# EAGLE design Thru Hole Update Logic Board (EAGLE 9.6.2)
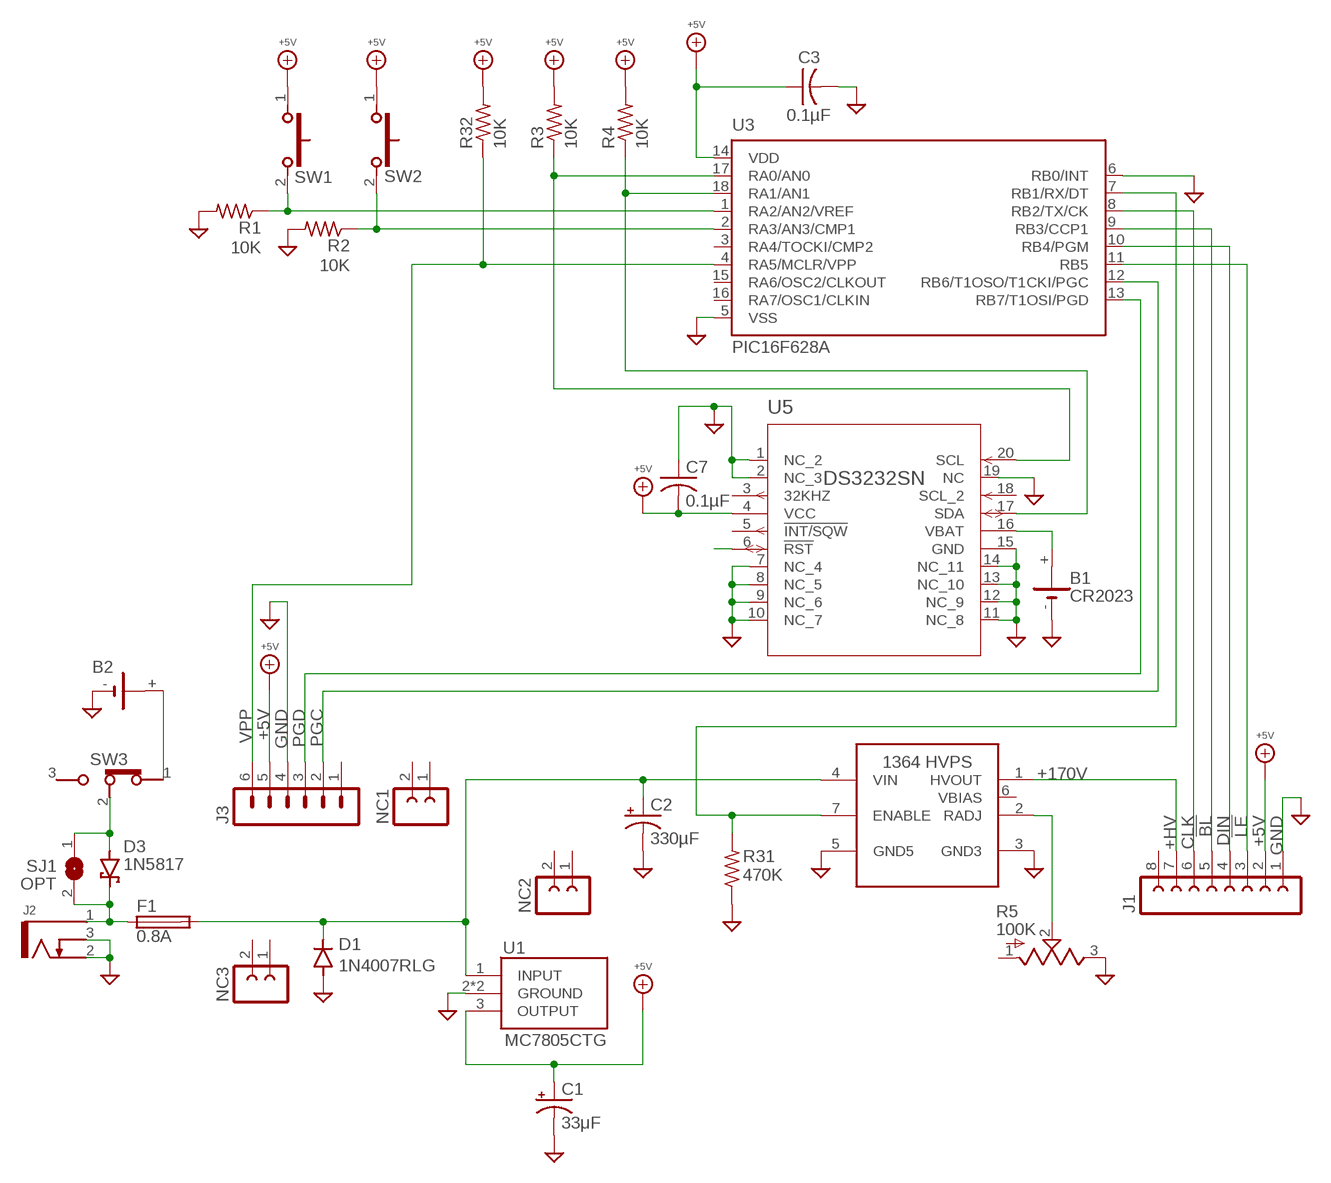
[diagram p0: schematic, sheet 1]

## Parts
B1  CR2023  BATTERY  [103]
B2  BATTERYWIRE_ATTACH  BATTERY1291  [1291]
C1  33μF  CPOL-USE2-5  [E2-5]
C2  330µF  CPOL-USE3.5-8  [E3,5-8]
C3  0.1µF  C-US  [C025-040X050]
C7  0.1µF  C-USC0805  [C0805]
D1  1N4007RLG  RECTIFIER  [DO41-7]
D3  1N5817  SCHOTTKY  [DO41-7]
F1  0.8A  FUSE  [5X20MM]
J1  FE08  [FE08]
J2  KLDX-0202-B  [KDLX-0202-X]
J3  MA06  [MA06]
NC1  FE02  [FE02]
NC2  FE02  [FE02]
NC3  FE02  [FE02]
R1  10K  R-US0207/10  [0207/10]
R2  10K  R-US0207/10  [0207/10]
R3  10K  R-US0207/10  [0207/10]
R4  10K  R-US0207/10  [0207/10]
R5  100K  R-US_TRIM  [PV37W]
R31  470K  R-US0207/10  [0207/10]
R32  10K  R-US0207/10  [0207/10]
SJ1  OPT  SJ  [SJ]
SW1  FSMRA4JH04  SWITCH_PUSH_SPST_(ON)  [FSMRA4JH]
SW2  FSMRA4JH04  SWITCH_PUSH_SPST_(ON)  [FSMRA4JH]
SW3  5MS1S102AM6QES  SWITCH_SLIDE_SPDT_ON  [SLIDE_SPDT_MINI]
U1  MC7805CTG  [TO-220-3_RA]
U2  1364-HVPS-H  [1364-HVPS-H]
U3  PIC16F628A  PIC16F628P  [DIP-18]
U5  DS3232SN  [SOIC-20]

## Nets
!BL!: J1.5 U3.9(RB3/CCP1)
!LE!: J1.3 U3.11(RB5)
+5V: C1.+ C3.1 C7.2 J1.2 J3.5 R3.2 R4.2 R32.2 SW1.1 SW2.1 U1.3(OUTPUT) U3.14(VDD) U5.4(VCC)
+9V: D3.C F1.1A F1.1B J2.1 SJ1.2
+9V_1: C2.+ D1.C F1.2A F1.2B U1.1(INPUT) U2.4(VIN)
+9V_2: D3.A SJ1.1 SW3.2(COM)
+9V_4: B2.+ SW3.1(POS_1)
+HV: J1.7 U2.1(HVOUT)
BAT: B1.+ U5.16(VBAT)
CLK: J1.6 U3.8(RB2/TX/CK)
DIN: J1.4 U3.10(RB4/PGM)
ENABLE: R31.2 U2.7(ENABLE) U3.7(RB1/RX/DT)
GND: B1.- B2.- C1.- C2.- C3.2 C7.1 D1.A J1.1 J2.2 J2.3 J3.4 R1.2 R2.2 R5.3 R31.1 U1.2(GROUND) U1.2_1(GROUND) U2.3(GND3) U2.5(GND5) U3.5(VSS) U3.6(RB0/INT) U5.1(NC_2) U5.2(NC_3) U5.7(NC_4) U5.8(NC_5) U5.9(NC_6) U5.10(NC_7) U5.11(NC_8) U5.12(NC_9) U5.13(NC_10) U5.14(NC_11) U5.15(GND) U5.19(NC)
MYSTERY_3: U5.6(!RST)
PGC: J3.2 U3.12(RB6/T1OSO/T1CKI/PGC)
PGD: J3.3 U3.13(RB7/T1OSI/PGD)
RADJ: R5.2 U2.2(RADJ)
SCL: R3.1 U3.17(RA0/AN0) U5.20(SCL)
SDA: R4.1 U3.18(RA1/AN1) U5.17(SDA)
SW1: R1.1 SW1.2 U3.1(RA2/AN2/VREF)
SW2: R2.1 SW2.2 U3.2(RA3/AN3/CMP1)
VPP: J3.6 R32.1 U3.4(RA5/MCLR/VPP)
Unconnected: J1.8 J3.1 NC1.1 NC1.2 NC2.1 NC2.2 NC3.1 NC3.2 R5.1 SW3.3(POS_2) U2.6(VBIAS) U3.3(RA4/TOCKI/CMP2) U3.15(RA6/OSC2/CLKOUT) U3.16(RA7/OSC1/CLKIN) U5.3(32KHZ) U5.5(!INT/SQW) U5.18(SCL_2)

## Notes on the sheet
- +170V

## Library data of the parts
B1 B2 = My Imported Components:BATTERY: LI BATTERY Varta
C1 C2 = My Imported Components:CPOL-US
C3 = My Imported Components:C-US
C7 = rcl:C-US: CAPACITOR, American symbol; SPICEPREFIX: C
D1 = My Imported Components:RECTIFIER
D3 = My Imported Components:SCHOTTKY
F1 = My Imported Components:FUSE
J1 = My Imported Components:FE08: FEMALE HEADER; OC_FARNELL: unknown; OC_NEWARK: unknown
J2 = My Imported Components:KLDX-0202-B: https://www.mouser.com/datasheet/2/222/KLDX_0202-334781.pdf
J3 = My Imported Components:MA06: PIN HEADER; OC_FARNELL: unknown; OC_NEWARK: unknown
NC1-NC3 = My Imported Components:FE02: FEMALE HEADER
R1-R4 R31 R32 = My Imported Components:R-US: RESISTOR, American symbol; SPICEPREFIX: R
R5 = My Imported Components:R-US_TRIM: Res Cermet Trimmer 1M Ohm 10% 1/4W 12(Elec)Turn 1.8mm (6.4 X 4 X 7.7mm) Pin Thru-Hole Bulk Check prices; AVAILABILITY: Good; DESCRIPTION: 100 kOhms 0.25W, 1/4W PC Pins Through Hole Trimmer Potentiometer Cermet 12 Turn Top Adjustment; MF: Bourns; MP: PV37W104C01B00; PACKAGE: 3224X Bourns; PRICE: None; PURCHASE-URL: https://pricing.snapeda.com/search/part/PV37W104C01B00/?ref=eda
SJ1 = jumper:SJ: SMD solder JUMPER
SW1 SW2 = My Imported Components:SWITCH_PUSH_SPST_(ON)
SW3 = My Imported Components:SWITCH_SLIDE_SPDT_ON
U1 = My Imported Components:MC7805CTG: Voltage regulator,MC7805CT 5V 1A ON Semiconductor MC7805CTG, Single Linear Voltage Regulator, 1A 5 V, +/-4%, 3-Pin TO-220 Source: Datasheet; ARROW_PART_NUMBER: MC7805CTG; ARROW_PRICE-STOCK: https://www.arrow.com/en/products/mc7805ctg/on-semiconductor; DESCRIPTION: Voltage regulator,MC7805CT 5V 1A ON Semiconductor MC7805CTG, Single Linear Voltage Regulator, 1A 5 V, +/-4%, 3-Pin TO-220; HEIGHT: 4.82mm; MANUFACTURER_NAME: ON Semiconductor; MANUFACTURER_PART_NUMBER: MC7805CTG; MOUSER_PART_NUMBER: 863-MC7805CTG; MOUSER_PRICE-STOCK: https://www.mouser.co.uk/ProductDetail/ON-Semiconductor/MC7805CTG/?qs=%252B9%2Fcbd0IE0SRQQJXyw%252B9hQ%3D%3D
U2 = My Imported Components:1364-HVPS-H: https://www.shop-tes.com/content/Datasheets/8002K.pdf
U3 = My Imported Components:PIC16F62*: FLASH-Based 8-Bit CMOS Microcontroller Source: http://ww1.microchip.com/downloads/en/DeviceDoc/40300C.pdf; MF: MICROCHIP; MPN: PIC16F628-04I/P; OC_FARNELL: 9760407; OC_NEWARK: 19C7272
U5 = My Imported Components:DS3232SN; BUILT_BY: EMA_UL_Team; MANUFACTURER_PART_NUMBER: ds3232sn#; SOURCELIBRARY: Maxim_2009-12-17_1; VENDOR: Maxim Integrated Products

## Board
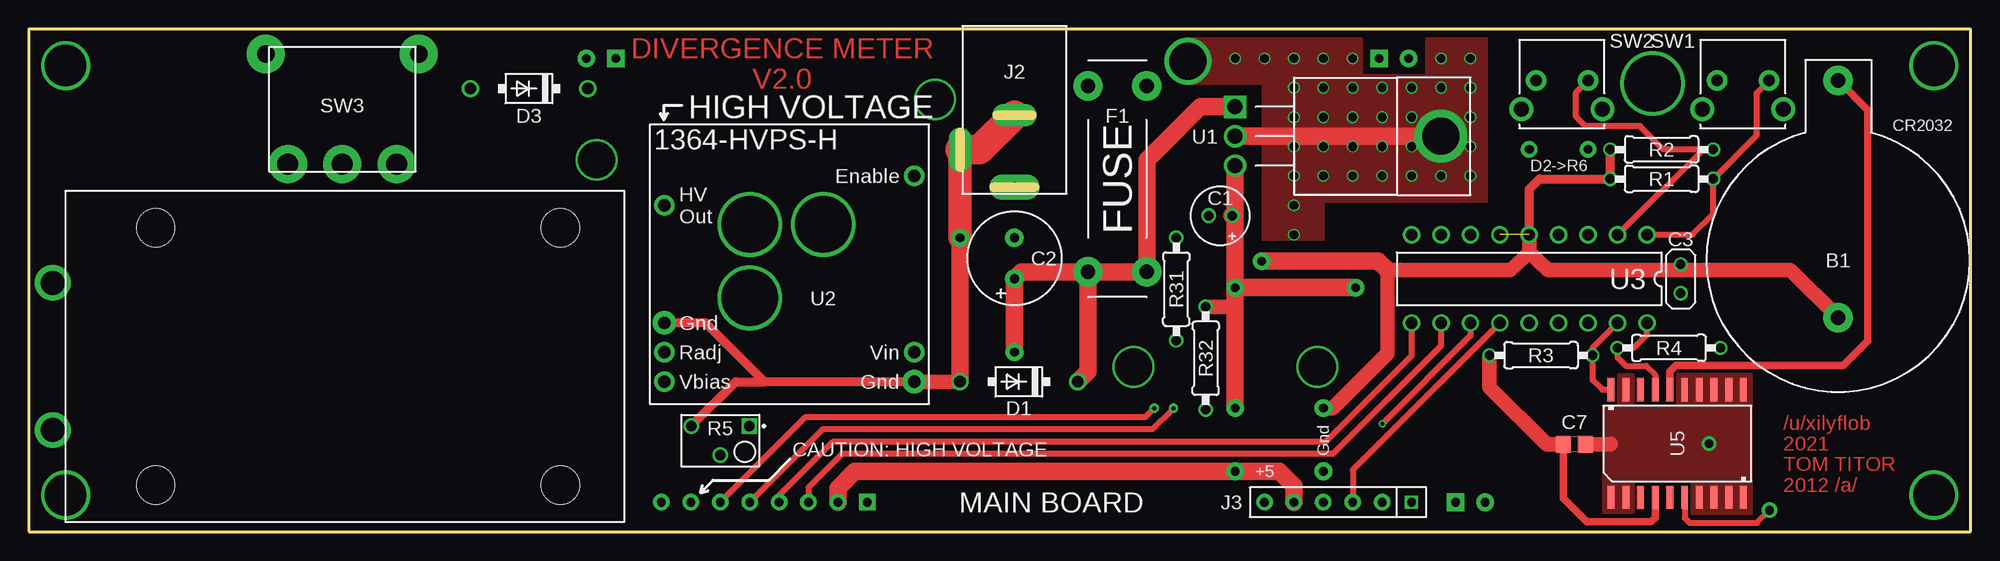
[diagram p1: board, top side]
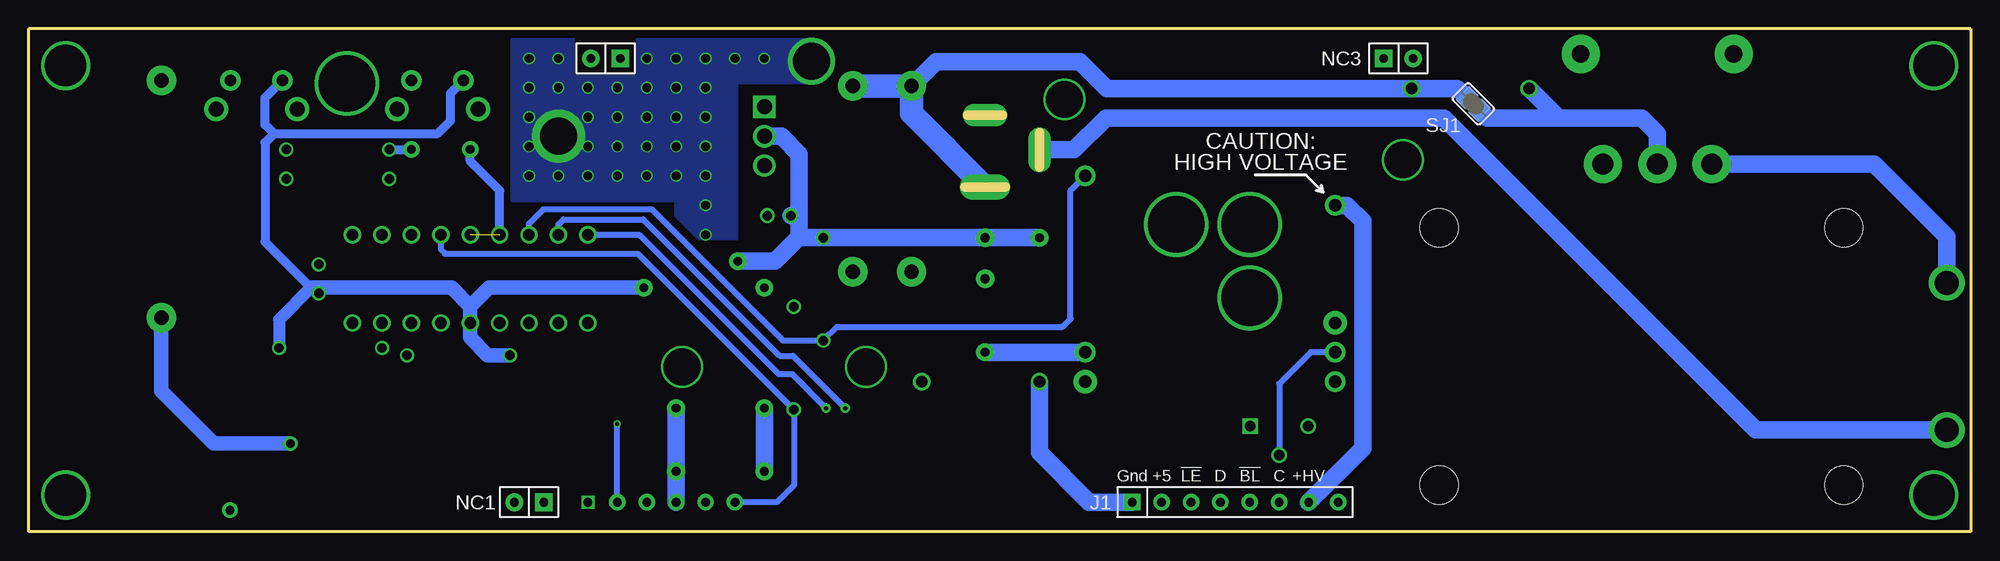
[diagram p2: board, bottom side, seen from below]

Size 167.64 x 43.43 mm. Coordinates in mm from the lower left corner, seen from the top.
Outline: 0,0 167.64,0 167.64,43.43 0,43.43 0,0
Copper layers (1*16): Top 0.035559375mm / dielectric 1.6mm / Bottom 0.035559375mm
Design rules "oshpark-2layer *": minimum track width 6mil, minimum drill 10mil, track to track 6mil, track to pad 6mil, pad to pad 6mil, via to via 6mil, smd to smd 6mil, copper to edge 15mil, drill to drill 6mil, minimum pad ring 5mil, minimum via ring 5mil, stop-mask expansion 2.5mil, vias tented up to drill 0mil, thermal gap 10mil

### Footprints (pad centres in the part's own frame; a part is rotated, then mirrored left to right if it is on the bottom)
103 = drill 1.27 pad 2.54: + 0,0; - 0,-20.498
1291 = drill 2.057: + 8.89,-6.35; - 8.89,6.35 | hole 3.302: -34.925,11.113; 0,11.113; 0,-11.113; -34.925,-11.113
E2-5 = drill 0.813 pad 1.27: + -1.016,0; - 1.016,0
E3,5-8 = drill 0.813 pad 1.6: + -1.778,0; - 1.778,0
C025-040X050 = drill 0.813: 1 -1.25,0; 2 1.25,0
C0805 = smd 1.3 x 1.5: 1 -0.95,0; 2 0.95,0
DO41-7 = drill 1: A 5.08,0; C -5.08,0
5X20MM = drill 1.245 pad 2.54: 1A -8.026,2.54; 1B -8.026,-2.54; 2A 8.026,2.54; 2B 8.026,-2.54
FE08 = drill 0.75 pad 1.422 square: 1 -8.89,0 | drill 0.75 pad 1.422: 2 -6.35,0; 3 -3.81,0; 4 -1.27,0; 5 1.27,0; 6 3.81,0; 7 6.35,0; 8 8.89,0
KDLX-0202-X = drill 0.8 pad 2.184 long: 1 13.9,0 | drill 0.8 pad 1.93 long: 2 7.7,0; 3 10.7,-4.7
MA06 = drill 0.75 square: 1 -6.35,0 | drill 0.75 pad 1.422: 2 -3.81,0; 3 -1.27,0; 4 1.27,0; 5 3.81,0; 6 6.35,0
FE02 = drill 0.75 pad 1.524 square: 1 -1.27,0 | drill 0.75 pad 1.524: 2 1.27,0
0207/10 = drill 0.813: 1 -4.445,0; 2 4.445,0
PV37W = drill 0.9 square: 1 -2.5,-1.25 | drill 0.9: 2 0,1.25; 3 2.5,-1.25
SJ = smd 1.168 x 1.6: 1 -0.762,0; 2 0.762,0
FSMRA4JH = drill 0.991 pad 1.753: 1 4.496,0; 2 0,0 | drill 1.295 pad 2.057: 3 -1.245,2.489; 4 5.766,2.489
SLIDE_SPDT_MINI = drill 1.8 pad 3.302: 1 -4.699,0; 2 0,0; 3 4.699,0 | drill 1.5 pad 3.302: P$4 -6.604,9.525; P$5 6.604,9.525
TO-220-3_RA = drill 1.29 pad 1.935 square: 1 0,0 | drill 1.29 pad 1.935: 2 2.54,0; 3 5.08,0 | drill 3.175 pad 4.572: 2_1 2.54,17.78
1364-HVPS-H = drill 1.067 pad 1.778: 1 1.27,17.145; 2 1.27,4.445; 4 22.86,4.445; 6 1.27,1.905; 7 22.86,19.685 | drill 1.067 pad 2.032: 3 1.27,6.985; 5 22.86,1.905
DIP-18 = drill 1: 1 -10.16,-3.81; 2 -7.62,-3.81; 3 -5.08,-3.81; 4 -2.54,-3.81; 5 0,-3.81; 6 2.54,-3.81; 7 5.08,-3.81; 8 7.62,-3.81; 9 10.16,-3.81; 10 10.16,3.81; 11 7.62,3.81; 12 5.08,3.81; 13 2.54,3.81; 14 0,3.81; 15 -2.54,3.81; 16 -5.08,3.81; 17 -7.62,3.81; 18 -10.16,3.81
SOIC-20 = smd 2 x 0.6: 1 -4.65,5.715; 2 -4.65,4.445; 3 -4.65,3.175; 4 -4.65,1.905; 5 -4.65,0.635; 6 -4.65,-0.635; 7 -4.65,-1.905; 8 -4.65,-3.175; 9 -4.65,-4.445; 10 -4.65,-5.715; 11 4.65,-5.715; 12 4.65,-4.445; 13 4.65,-3.175; 14 4.65,-1.905; 15 4.65,-0.635; 16 4.65,0.635; 17 4.65,1.905; 18 4.65,3.175; 19 4.65,4.445; 20 4.65,5.715

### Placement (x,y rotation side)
B1  156.21,38.99 0 top
B2  10.95,15.14 180 top
C1  102.87,27.3 180 top
C2  85.09,23.62 90 top
C3  142.62,21.84 90 top
C7  133.44,7.54 180 top
D1  85.47,12.95 180 top
D3  43.18,38.28 180 top
F1  93.98,30.48 270 top
J1  63.5,2.54 0 bottom
J2  85.09,43.69 270 top
J3  113.03,2.54 180 top
NC1  124.46,2.54 180 bottom
NC2  117.86,40.89 180 bottom
NC3  49.4,40.89 0 bottom
R1  140.97,30.48 180 top
R2  140.97,33.02 180 top
R3  130.56,15.24 180 top
R4  141.6,15.88 0 top
R5  59.69,7.87 180 top
R31  99.06,20.95 270 top
R32  101.6,14.99 90 top
SJ1  42.93,36.96 135 bottom
SW1  150.24,38.99 180 top
SW2  134.62,38.99 180 top
SW3  27.05,31.75 0 top
U1  104.14,36.7 270 top
U2  53.59,11.05 0 top
U3  129.54,21.84 180 top
U5  142.32,7.62 90 top

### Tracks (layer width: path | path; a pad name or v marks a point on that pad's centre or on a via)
!BL!  (via drill 0.35 pad 0.79)
  Top 0.508: J1.5 68.53,8.84 96.98,8.84 v98.81,10.67
  Bottom 0.508: U3.9 114.96,25.65 102.89,13.59 101.73,13.59 v98.81,10.67
!LE!
  Top 0.508: U3.11 121.92,16.05 112.57,6.71 70.21,6.71 67.31,3.81 J1.3
+5V  (via drill 0.75 pad 1.52)
  Top 0.635: C7.2 132.49,2.89 134.52,0.86 140.06,0.86 140.41,1.22 U5.4
  Top 1.27: R32.2 104.06,19.43 104.14,19.36 | R3.2 126.11,12.47 131.04,7.54 C7.2
  Top 1.524: U1.3 104.14,27.2 | 104.14,27.2 v104.14,21.08 | v104.14,21.08 104.14,19.36 v104.14,10.67 | J1.2 69.85,3.76 71.3,5.21 v104.14,5.21 107.97,5.21 109.22,3.96 J3.5 | C1.+ 104.11,27.23 104.14,27.2 | v104.14,21.08 v114.55,21.08
  Bottom 0.762: 146.47,34.39 132.36,34.39 131.24,35.51 131.24,37.87 SW2.1 | 146.47,34.39 147.24,33.62 147.24,25.03 143.3,21.08 | 146.47,34.39 147.24,35.16 147.24,37.49 SW1.1
  Bottom 1.016: 143.3,21.08 146.05,18.33 R4.2
  Bottom 1.27: v114.55,21.08 127.91,21.08 129.54,19.46 | 129.54,19.46 U3.14 129.54,16.76 128.02,15.24 R3.2 | 142.62,21.08 131.17,21.08 129.54,19.46 | 142.62,21.08 143.3,21.08 | C3.1 142.62,21.08
  Bottom 1.524: v104.14,10.67 v104.14,5.21
+9V
  Bottom 1.016: 43.71,37.69 43.49,37.47 SJ1.2
  Bottom 1.524: F1.1B 89.33,40.62 76.91,40.62 74.57,38.28 D3.C 44.3,38.28 43.71,37.69
  Bottom 2.032: J2.1 91.44,36.14 F1.1B F1.1A
+9V_1  (via drill 0.75 pad 1.52)
  Top 1.524: F1.2B F1.2A 96.52,32.08 101.14,36.7 U1.1 | F1.2B 85.7,22.45 C2.+ v85.09,15.49 | F1.2B 91.44,13.84 D1.C
  Bottom 1.524: U2.4 v85.09,15.49
+9V_2
  Bottom 1.016: SJ1.1 42.41,36.39 42.11,36.09
  Bottom 1.524: SW3.2 27.05,34.39 28.37,35.71 35.53,35.71 | D3.A 35.53,35.71 | 42.11,36.09 41.73,35.71 35.53,35.71
+9V_4
  Bottom 1.524: B2.+ 2.06,25.48 8.33,31.75 SW3.1
+HV
  Bottom 1.524: U2.1 53.85,28.19 52.48,26.82 52.48,7.21 J1.7
BAT
  Top 0.635: B1.+ 158.78,36.42 158.78,16.48 156.67,14.38 142.22,14.38 141.68,13.84 U5.16
CLK  (via drill 0.35 pad 0.79)
  Top 0.508: v97.16,10.67 96.37,9.88 67.03,9.88 J1.6
  Bottom 0.508: U3.8 121.92,26.54 121.49,26.98 114.61,26.98 102.82,15.19 101.68,15.19 v97.16,10.67
DIN
  Top 0.508: U3.10 119.38,15.19 111.94,7.75 69.39,7.75 64.77,3.12 J1.4
ENABLE
  Bottom 0.508: U2.7 77.7,29.49 77.7,18.39 78.38,17.7 97.87,17.7 R31.2 102.51,16.51 113.87,27.86 123.22,27.86 124.46,26.62 U3.7
GND  (via drill 0.75, 0.75 pad 1.27, 0.75 pad 1.42, 0.75 pad 1.52, 3.17 pad 4.06)  (1 unrouted)
  Top 0.762: U2.3 58.44,18.03 63.52,12.95 | U3.5 129.54,29.59 130.43,30.48 R1.2 R2.2 | U2.5 63.52,12.95 | R5.3 61.02,12.95 63.52,12.95
  Top 1.27: D1.A U2.5 | 142.62,22.61 131.17,22.61 129.54,24.13 | U3.5 129.54,24.13 | 129.54,24.13 127.91,22.61 117.3,22.61 117.3,15.42 112.55,10.67 v111.76,10.67 | B1.- 152.09,22.61 142.62,22.61 | C7.1 136.53,7.54 136.58,7.59 | C3.2 142.62,22.61
  Top 1.524: v80.39,25.4 D1.A | v106.43,23.37 116.48,23.37 117.3,22.61 | U1.2 U1.2_1
  Top 2.032: J2.3 v80.39,25.4
  Top 2.54: J2.2 82.09,32.99 J2.3
  Bottom 0.762: U3.6 127,29.46 129.54,32 v129.54,33.02 | R2.2 v134.62,33.02
  Bottom 1.27: B1.- 156.21,12.14 151.69,7.62 v145.06,7.62
  Bottom 1.524: v80.39,25.4 C2.- R31.1 101.14,25.4 | J1.1 76.1,2.54 80.39,6.83 D1.A | 101.14,25.4 101.14,27.3 | 101.14,27.3 101.14,32.64 102.67,34.16 U1.2 | 101.14,25.4 101.19,25.4 103.23,23.37 v106.43,23.37 | C1.- 101.14,27.3 | v111.76,10.67 v111.76,5.21 J3.4 | J2.3 77.4,32.99 74.65,35.74 45.49,35.74 18.54,8.79 B2.-
  other vias: 104.14,40.89 106.68,40.89 109.22,40.89 111.76,40.89 114.3,40.89 109.22,38.35 111.76,38.35 114.3,38.35 116.84,38.35 100.08,40.64 119.38,38.35 121.92,38.35 124.46,38.35 124.46,35.81 124.46,33.27 124.46,30.73 121.92,30.73 119.38,30.73 116.84,30.73 114.3,30.73 111.76,30.73 109.22,30.73 109.22,28.19 109.22,25.65 109.22,33.27 111.76,33.27 114.3,33.27 116.84,33.27 119.38,33.27 119.38,35.81 116.84,35.81 114.3,35.81 111.76,35.81 109.22,35.81 124.46,40.89 121.92,40.89
  pour Top (no thermals): 100.15,42.6 100.15,38.68 106.5,38.68 106.5,25.22 111.81,25.22 111.81,28.52 125.91,28.52 125.91,42.6 120.6,42.6 120.6,39.42 115.11,39.42 115.11,42.6
  pour Bottom (no thermals): 100.15,42.6 100.15,38.68 106.5,38.68 106.5,25.22 109.8,25.22 111.81,27.23 111.81,28.52 125.91,28.52 125.91,42.6 120.6,42.6 120.6,39.42 115.11,39.42 115.11,42.6
  pour Top (no thermals): 148.72,13.67 148.72,1.5 143.59,1.5 143.59,4.37 138.51,4.37 138.51,1.63 135.92,1.63 135.92,10.9 137.24,10.9 137.24,13.61 138.51,13.61 138.51,10.9 142.32,10.9 142.32,13.67
MYSTERY_3  (via drill 0.75 pad 1.35)
  Top 0.508: U5.6 142.95,1.19 143.38,0.76 149.2,0.76 v150.29,1.85
N$3  (via drill 3.17 pad 3.61)
  other vias: 49.02,32.13
N$21  (via drill 3.58 pad 4.27)
  other vias: 3.17,40.26
N$22  (via drill 3.58 pad 4.27)
  other vias: 3.17,3.17
N$23  (via drill 3.58 pad 4.27)
  other vias: 164.47,40.26
N$24  (via drill 3.58 pad 4.27)
  other vias: 164.47,3.17
N$25  (via drill 3.17 pad 3.61)
  other vias: 78.23,37.34
N$26  (via drill 3.17 pad 3.61)
  other vias: 95.38,14.22
N$27  (via drill 3.17 pad 3.61)
  other vias: 111.25,14.22
N$28  (via drill 4.88 pad 5.59)
  other vias: 62.23,26.54
N$29  (via drill 4.88 pad 5.59)
  other vias: 68.58,26.54
N$30  (via drill 4.88 pad 5.59)
  other vias: 62.23,20.19
N$31  (via drill 4.88 pad 5.59)
  other vias: 140.18,38.73
PGC  (via drill 0.35)
  Top 0.508: U3.12 124.46,16.94 v116.84,9.32
  Bottom 0.508: J3.2 v116.84,9.32
PGD
  Top 0.508: J3.3 114.3,5.33 U3.13
RADJ
  Bottom 0.508: U2.2 56.97,15.49 59.69,12.78 R5.2
SCL
  Top 0.508: U3.17 135,15.88 R3.1 135,13.11 135.84,12.27 U5.20
SDA
  Top 0.508: U3.18 139.7,16.99 138.58,15.88 R4.1 137.16,15.04 137.87,14.33 139.62,14.33 140.41,13.54 U5.17
SW1
  Top 0.508: U3.1 143.64,25.65 145.41,27.43 R1.1 149.17,34.24 149.17,37.92 SW1.2
SW2
  Top 0.508: 144.55,33.02 137.19,25.65 U3.2 | SW2.2 133.58,37.95 133.58,35.84 134.37,35.05 139.09,35.05 141.12,33.02 144.55,33.02 | R2.1 144.55,33.02
VPP
  Bottom 0.508: U3.4 132.08,24.38 131.72,24.03 115.09,24.03 R32.1 101.6,3.99 103.05,2.54 J3.6

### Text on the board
Top: DIVERGENCE METER / V2.0 | /u/xilyflob / 2021 / TOM TITOR / 2012 /a/
tPlace: HIGH VOLTAGE | CR2032 | D2->R6 | Gnd | CAUTION: HIGH VOLTAGE | +5 | MAIN BOARD
bPlace: CAUTION: / HIGH VOLTAGE | +HV | C | !BL! | D | !LE! | +5 | Gnd
tStop: DIVERGENCE METER / V2.0 | /u/xilyflob / 2021 / TOM TITOR / 2012 /a/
